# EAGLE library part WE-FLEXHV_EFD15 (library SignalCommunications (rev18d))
WE-FLEX HV Flexible Transformer for DC/DC Converter Characteristics Transformer with 6 identical windings 4 sizes with 5 different lengths of air gap each Isolation voltage up to 1.5 kVAC Low leakage inductance Operating temperature: –40 ºC to +125 ºC By using different circuits more than 375 transformer solutions and about 125 choke solutions possible. Consequently, quick prototyping possibilities EFD size parts provide Basic insulation for a working voltage of 250VRMS when they are connteced approbiate Applications Flyback converters Forward converters Push-pull converters Step-up/step-down converters SEPIC Details see: http://katalog.we-online.de/en/pbs/WE-FLEXHV/749196308?m Created by Yingchun Shan 2017 (C) Wurth Elektronik
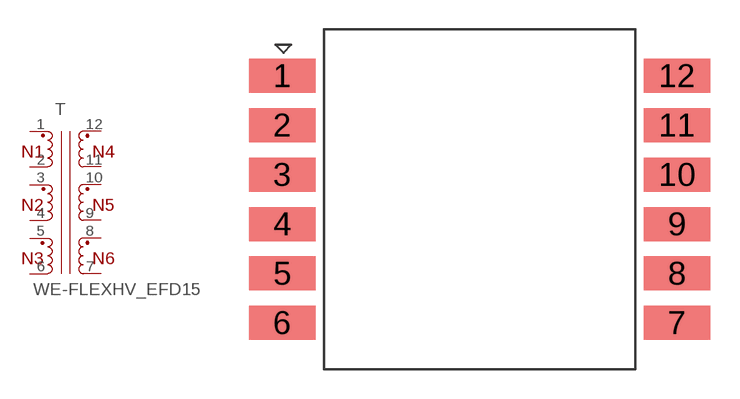
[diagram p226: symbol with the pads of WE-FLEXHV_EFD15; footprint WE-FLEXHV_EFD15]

Designator prefix T

## WE-FLEXHV_EFD15_749196308 (WE-NUMBER: 749196308/153,8uH), WE-FLEXHV_EFD15_749196318 (WE-NUMBER: 749496318/23,3uH), WE-FLEXHV_EFD15_749196328 (WE-NUMBER: 749196328/14,2uH), WE-FLEXHV_EFD15_749196338 (WE-NUMBER: 749496338/9,3uH), WE-FLEXHV_EFD15_749196348 (WE-NUMBER: 749196348/7,9uH)  [WE-FLEXHV_EFD15]
1  1  pas
2  2  pas
3  3  pas
4  4  pas
5  5  pas
6  6  pas
7  7  pas
8  8  pas
9  9  pas
10  10  pas
11  11  pas
12  12  pas

## Footprint WE-FLEXHV_EFD15 (pad centres in mm)
smd 3.43 x 1.75: 1 -10.155,6.35; 2 -10.155,3.81; 3 -10.155,1.27; 4 -10.155,-1.27; 5 -10.155,-3.81; 6 -10.155,-6.35; 7 10.155,-6.35; 8 10.155,-3.81; 9 10.155,-1.27; 10 10.155,1.27; 11 10.155,3.81; 12 10.155,6.35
